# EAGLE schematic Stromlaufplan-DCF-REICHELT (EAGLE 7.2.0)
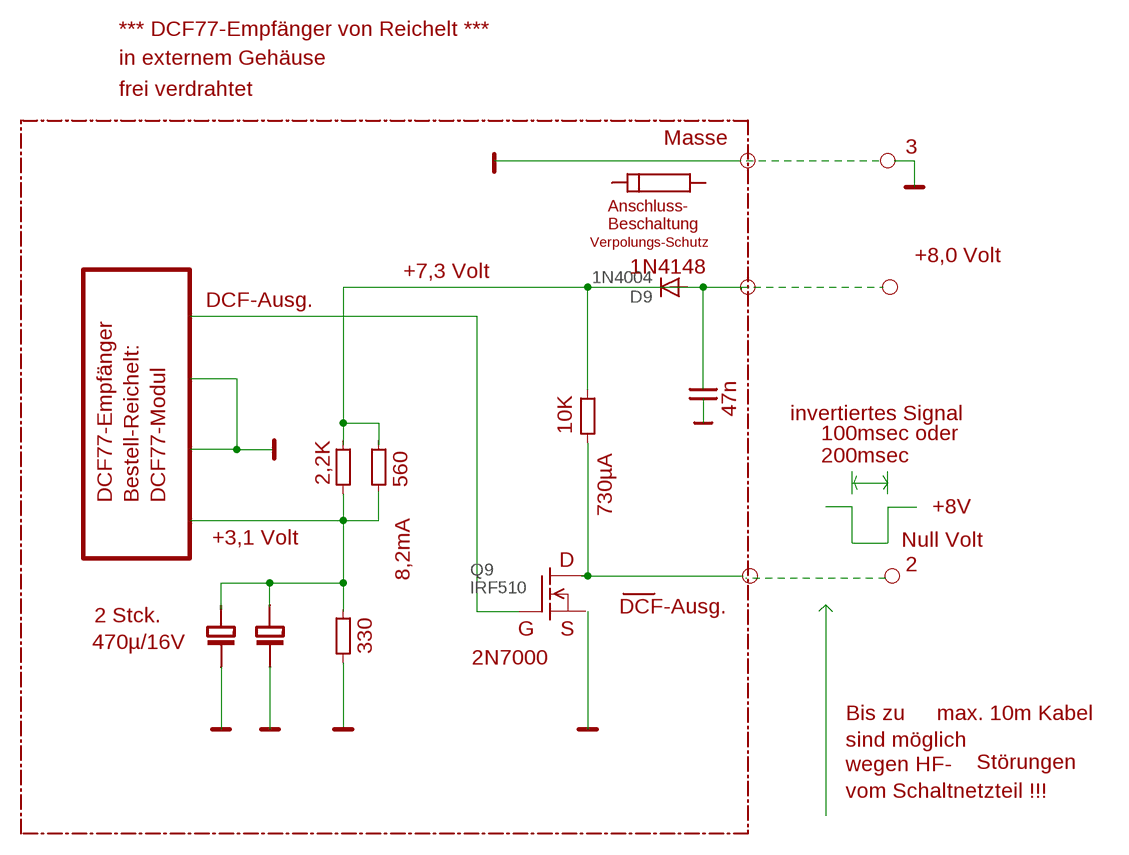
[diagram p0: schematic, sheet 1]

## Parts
D9  1N4004  [DO41-10]
Q9  IRF510  [TO220]

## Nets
N$197: Q9.2(D)
N$210: Q9.1(G)
N$217: D9.A D9.C
Unconnected: Q9.3(S)

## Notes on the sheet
- *** DCF77-Empfänger von Reichelt ***
- in externem Gehäuse
- frei verdrahtet
- Masse
- 3
- Anschluss-
- Beschaltung
- Verpolungs-Schutz | +8,0 Volt
- +7,3 Volt | 1N4148
- DCF-Ausg.
- 47n
- invertiertes Signal
- 10K
- 100msec oder
- 200msec
- 2,2K | 560
- DCF77-Empfänger | Bestell-Reichelt: | DCF77-Modul
- 730µA | +8V
- +3,1 Volt | Null Volt
- D | 2
- 8,2mA
- DCF-Ausg.
- 2 Stck.
- G | S
- 470µ/16V | 330
- 2N7000
- Bis zu | max. 10m Kabel
- sind möglich
- wegen HF- | Störungen
- vom Schaltnetzteil !!!

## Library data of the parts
D9 = diode:1N4004: DIODE
Q9 = transistor-fet:IRF510: N-Channel Enhancement MOSFET (HEXFET); 100V; 5,6A; 0,54Ohm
